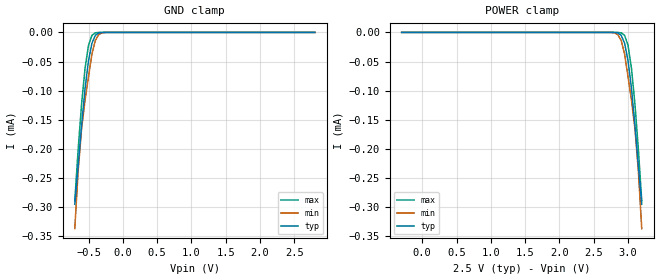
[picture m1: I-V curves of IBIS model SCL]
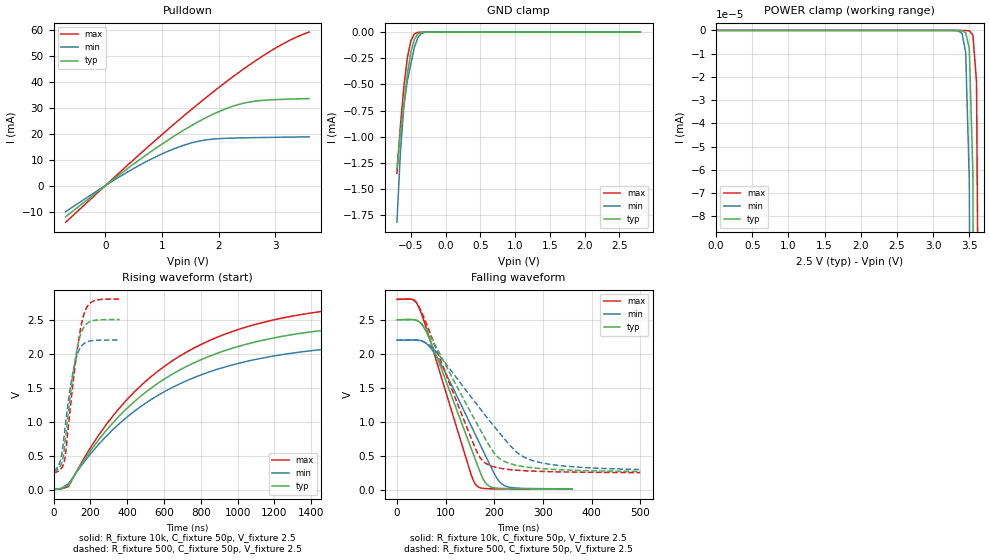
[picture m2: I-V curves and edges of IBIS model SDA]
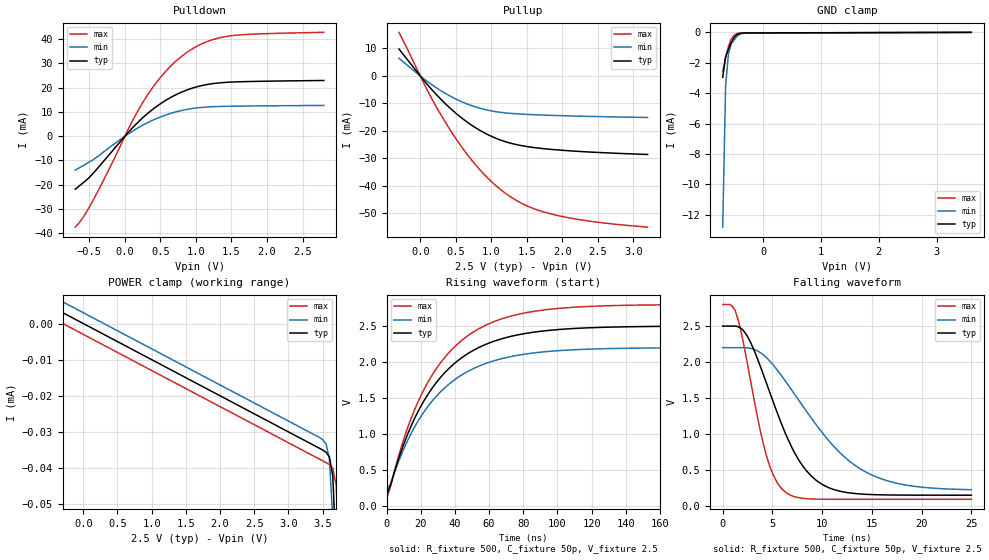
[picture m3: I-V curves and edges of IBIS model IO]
| PCA9538 - IBIS model
[IBIS Ver]   3.2
[Comment Char]   |_char
| VDD nom: 2.5v; min: 2.2v; max: 2.8v
[File name]   pca9538_2_5v.ibs
[File Rev]   1
[Date]   Aug 18, 2008 11:26:38 AM
[Source]
[Notes]
[Disclaimer]
(C) Copyright 2007 NXP Semiconductors
All rights reserved
NXP Semiconductors (NXP) does not warrant that this model and any other
accompanying information (Model) accurately or fully represents the
operating characteristics and specifications of the semiconductor
products to which the Model relates.  Moreover, the Model is furnished
on an "as is" and with "all faults" basis, and without support or
warranty of any kind.  NXP disclaims all warranties, whether expressed
or implied or statutory, including without limitation all implied
warranties of non-infringement, merchantability and fitness for any
purpose, and those arising from a course of dealing or usage of trade.
NXP does not convey any license under its or any third party's patents,
copyrights or other intellectual property or proprietary rights.
You and your company assume any and all risks and liability arising out
of the application or use of the Model.
In no event shall NXP be liable for any direct, indirect, special,
consequential or incidental damages, however caused, whether in
warranty, contract or tort (including negligence), strict liability or
other legal theory, including, without limitation, for lost profits,
business interruption, or corruption or loss of data or information,
arising out of or in connection with the use of or the inability to use
the Model, even if NXP has been advised of the possibility of such
damages.
NXP provides the Model as a courtesy to our customers. You and your
company shall not distribute, convey, sell, or give the Model to anyone
else without receiving prior written permission from NXP.
NXP reserves the right to make changes without notice to the Model to
improve reliability, function, or design.
Please be aware that your receipt and subsequent use of the Model shall
serve as acceptance of these terms and conditions.  If you do not
accept these terms, return or destroy the Model immediately.
[Copyright]
2008
| TSSOP16
[Component]   PCA9633PW
Si_location Pin
Timing_location Pin
[Manufacturer]   NXP Semiconductors
[Package]
R_pkg   3.92e-02   3.52e-02   4.56e-02
L_pkg   1.94n   1.65n   2.4n
C_pkg   0.446p   0.335p   0.771p
[Pin] signal_name   model_name   R_pin   L_pin   C_pin
1   A0   Addr   3.52E-02  2.40E-09  0.436E-12
2   A1   Addr   3.70E-02  1.93E-09  0.438E-12
3   RESETb   RESETb   4.56E-02  1.76E-09  0.345E-12
4   IO0   IO   4.00E-02  1.65E-09  0.335E-12
5   IO1   IO   4.00E-02  1.65E-09  0.335E-12
6   IO2   IO   4.56E-02  1.76E-09  0.345E-12
7   IO3   IO   3.70E-02  1.93E-09  0.438E-12
8   Vss   GND   3.52E-02  2.40E-09  0.452E-12
9   IO4   IO   3.52E-02  2.40E-09  0.452E-12
10   IO5   IO   3.70E-02  1.93E-09  0.438E-12
11   IO6   IO   4.56E-02  1.76E-09  0.345E-12
12   IO7   IO   4.00E-02  1.65E-09  0.771E-12
13   INTb   INT_OUT   4.00E-02  1.65E-09  0.771E-12
14   SCL   SCL   4.56E-02  1.76E-09  0.345E-12
15   SDA   SDA   3.70E-02  1.93E-09  0.438E-12
16   VDD   POWER   3.52E-02  2.40E-09  0.452E-12
| SO16
[Component]   PCA9633D16
Si_location Pin
Timing_location Pin
[Manufacturer]   NXP Semiconductors
[Package]
R_pkg   4.96e-02   3.94e-02   5.98e-02
L_pkg   2.52n   1.87n   3.16n
C_pkg   0.628p   0.494p   0.763p
[Pin] signal_name   model_name   R_pin   L_pin   C_pin
1   A0   Addr   5.98E-02  3.16E-09  7.63E-13
2   A1   Addr   4.55E-02  2.41E-09  6.04E-13
3   RESETb   RESETb   4.64E-02  1.93E-09  5.15E-13
4   IO0   IO   3.94E-02  1.87E-09  4.94E-13
5   IO1   IO   3.94E-02  1.87E-09  4.94E-13
6   IO2   IO   4.64E-02  1.93E-09  5.15E-13
7   IO3   IO   4.55E-02  2.41E-09  6.04E-13
8   Vss   GND   5.98E-02  3.16E-09  7.63E-13
9   IO4   IO   5.98E-02  3.16E-09  7.63E-13
10   IO5   IO   4.55E-02  2.41E-09  6.04E-13
11   IO6   IO   4.64E-02  1.93E-09  5.15E-13
12   IO7   IO   3.94E-02  1.87E-09  4.94E-13
13   INTb   INT_OUT   3.94E-02  1.87E-09  4.94E-13
14   SCL   SCL   4.64E-02  1.93E-09  5.15E-13
15   SDA   SDA   4.55E-02  2.41E-09  6.04E-13
16   VDD   POWER   5.98E-02  3.16E-09  7.63E-13
[Define Package Model]  HVQFN16
[Manufacturer]  ST-NXP Wireless
[OEM]  Unknown
[Description]  Full package model
|[Simulated] Chris Hunat
|[Approved] Wayne Nunn, Roger Real
[Number Of Pins]  16
[Pin Numbers]
|Pin Num   Terminal Name
1   | lead1:pin1
2   | lead2:pin2
3   | lead3:pin3
4   | lead4:pin4
5   | lead5:pin5
6   | lead6:pin6
7   | lead7:pin7
8   | lead8:pin8
9   | lead9:pin9
10   | lead10:pin10
11   | lead11:pin11
12   | lead12:pin12
13   | lead13:pin13
14   | lead14:pin14
15   | lead15:pin15
16   | lead16:pin16
[Model Data]
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[End Model Data]
[End Package Model]
| Models and submodels in the file (6): SCL (Input), SDA (I/O_open_drain), IO (I/O), RESETb (Input), INT_OUT (Open_drain), Addr (Input)
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[Model]   SCL
Model_type Input
Vinh=1.5
Vinl=0.75
C_comp   1.84p   1.81p   1.86p
[Temperature Range] 27   85   -40
[Voltage Range]   2.5   2.2   2.8
[GND Clamp]
-700mV    -295uA     -337uA     -289.5uA
-650mV    -228.6uA   -236.2uA   -199.5uA
-600mV    -158.8uA   -164.3uA   -122uA
-550mV    -96.13uA   -116.2uA   -61.46uA
-500mV    -48.62uA   -75.94uA   -22.35uA
-450mV    -18.67uA   -37.44uA   -5.001uA
-400mV    -4.926uA   -13.83uA   -710.6nA
-350mV    -920.5nA   -3.647uA   -77.67nA
-300mV    -138.4nA   -722.3nA   -7.551nA
-200mV    -2.42nA    -18.61nA   -62.47pA
2.8V      6.71pA     20.63pA    5.609pA
[POWER Clamp]
-300mV    6.71pA     20.63pA    5.609pA
2.7V      -2.42nA    -18.61nA   -62.47pA
2.8V      -138.4nA   -722.3nA   -7.551nA
2.85V     -920.5nA   -3.647uA   -77.68nA
2.9V      -4.926uA   -13.83uA   -710.6nA
2.95V     -18.67uA   -37.44uA   -5.001uA
3V        -48.62uA   -75.94uA   -22.35uA
3.05V     -96.13uA   -116.2uA   -61.46uA
3.1V      -158.8uA   -164.3uA   -122uA
3.15V     -228.6uA   -236.2uA   -199.5uA
3.2V      -295uA     -337uA     -289.5uA
[Model]   SDA
Model_type I/O_open_drain
Enable Active-High
Vinh=1.75
Vinl=0.75
Vref=2.5
Vmeas=1.25
Rref=10k
Cref=50p
C_comp   6.2p   6p   6.4p
[Temperature Range] 27   85   -40
[Voltage Range]   2.5   2.2   2.8
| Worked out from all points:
|   slope of the pulldown table from 0 to 0.375 V, typ, clamps not added: 59.7 ohm
|   GND clamp passes 1 mA (typ) near -0.65 V on its own axis
|   falling waveform, R_fixture 10k, C_fixture 50p, V_fixture 2.5: 20-80 % time 78.3ns typ, 88.6ns min, 71.3ns max; typ from 2.5 V to 0.016 V
|   falling waveform, R_fixture 500, C_fixture 50p, V_fixture 2.5: 20-80 % time 100ns typ, 125ns min, 83.5ns max; typ from 2.5 V to 0.275 V
|   rising waveform, R_fixture 10k, C_fixture 50p, V_fixture 2.5: 20-80 % time 701ns typ, 702ns min, 701ns max; typ from 0.015 V to 2.5 V
|   rising waveform, R_fixture 500, C_fixture 50p, V_fixture 2.5: 20-80 % time 63.7ns typ, 60.2ns min, 67.6ns max; typ from 0.265 V to 2.5 V
[Pulldown]
-700mV    -12mA      -10.04mA   -14.1mA
200mV     3.382mA    2.732mA    4.024mA
800mV     13.01mA    10.12mA    15.83mA
1.35V     20.92mA    15.31mA    26.22mA
1.6V      24.11mA    16.9mA     30.76mA
1.85V     26.97mA    17.83mA    35.17mA
2.2V      30.21mA    18.29mA    41.08mA
2.55V     32.25mA    18.47mA    46.6mA
2.85V     32.97mA    18.58mA    50.94mA
3.15V     33.27mA    18.68mA    54.79mA
3.4V      33.44mA    18.75mA    57.48mA
3.6V      33.55mA    18.8mA     59.2mA
[GND Clamp]
-700mV    -1.302mA   -1.818mA   -1.351mA
-650mV    -970uA     -1.147mA   -895.5uA
-600mV    -683.7uA   -711.2uA   -519.4uA
-550mV    -399.4uA   -467.3uA   -244.7uA
-500mV    -192.3uA   -305.3uA   -82.59uA
-450mV    -70.46uA   -146.9uA   -17.18uA
-400mV    -17.84uA   -52.38uA   -2.302uA
-350mV    -3.222uA   -13.43uA   -238.8nA
-300mV    -468.9nA   -2.601uA   -22.09nA
-200mV    -7.684nA   -64.03nA   -166.2pA
2.8V      13.86pA    54.83pA    11.22pA
[POWER Clamp]
0V        16.1pA     60.18pA    13.22pA
3.35V     -12.07pA   -161.9pA   -287.6fA
3.4V      -112.6pA   -1.322nA   -1.543pA
3.45V     -940.4pA   -9.345nA   -14.46pA
3.5V      -7.684nA   -64.03nA   -166.2pA
3.55V     -61.43nA   -424.5nA   -1.939nA
3.6V      -468.9nA   -2.601uA   -22.09nA
3.65V     -3.222uA   -13.43uA   -238.8nA
4V        -1.302mA   -1.818mA   -1.351mA
[Falling Waveform]
R_fixture=10k
C_fixture=50p
V_fixture=2.5
V_fixture_min=2.2
V_fixture_max=2.8
0s        2.5V       2.2V       2.8V
32.73ns   2.503V     2.203V     2.797V
47.27ns   2.46V      2.196V     2.646V
83.64ns   1.925V     1.936V     1.836V
152.7ns   607.1mV    940.1mV    222.7mV
163.6ns   400.2mV    777.2mV    65.93mV
185.5ns   80mV       453mV      21.86mV
207.3ns   27.97mV    155.1mV    18.26mV
221.8ns   23.24mV    63.63mV    17.19mV
360ns     16.11mV    18.89mV    14.52mV
[Falling Waveform]
R_fixture=500
C_fixture=50p
V_fixture=2.5
V_fixture_min=2.2
V_fixture_max=2.8
0s        2.5V       2.2V       2.8V
30.3ns    2.502V     2.202V     2.8V
45.45ns   2.473V     2.197V     2.691V
80.81ns   2.098V     2.027V     2.071V
161.6ns   1.01V      1.28V      606mV
181.8ns   749.8mV    1.095V     397mV
212.1ns   457.4mV    826.1mV    321.3mV
247.5ns   361.6mV    549.7mV    292mV
272.7ns   332.9mV    448.7mV    281.5mV
500ns     274.6mV    303.4mV    257.5mV
[Rising Waveform]
R_fixture=10k
C_fixture=50p
V_fixture=2.5
V_fixture_min=2.2
V_fixture_max=2.8
0s        14.58mV    15.74mV    13.8mV
80.81ns   70.46mV    91.25mV    51.11mV
202ns     580.6mV    534.6mV    627.3mV
323.2ns   988.5mV    888.1mV    1.089V
565.7ns   1.563V     1.386V     1.74V
808.1ns   1.919V     1.695V     2.143V
1.131us   2.193V     1.933V     2.453V
1.495us   2.35V      2.07V      2.631V
2.02us    2.447V     2.154V     2.74V
4us       2.498V     2.199V     2.798V
[Rising Waveform]
R_fixture=500
C_fixture=50p
V_fixture=2.5
V_fixture_min=2.2
V_fixture_max=2.8
0s        265.3mV    283.1mV    253.4mV
40ns      369.1mV    459mV      309.9mV
50.91ns   463.1mV    641.2mV    356.2mV
61.82ns   677.4mV    888.7mV    463.3mV
90.91ns   1.385V     1.494V     1.201V
120ns     1.948V     1.904V     1.881V
145.5ns   2.265V     2.085V     2.345V
170.9ns   2.412V     2.157V     2.622V
221.8ns   2.487V     2.194V     2.775V
360ns     2.5V       2.2V       2.8V
[Ramp]
R_load=500
dV/dt_r   1.769E+0/6.440E-8   1.721E+0/6.204E-8   1.801E+0/6.654E-8
dV/dt_f   1.737E+0/1.304E-7   1.574E+0/1.747E-7   1.791E+0/9.775E-8
|[End   SDA
[Model]   IO
Model_type I/O
Enable Active-High
Polarity Non-Inverting
Vinh=1.5
Vinl=0.75
Vref=2.5
Vmeas=1.25
Rref=500
Cref=50p
C_comp   8p   7.8p   8.2p
[Temperature Range] 27   85   -40
[Voltage Range]   2.5   2.2   2.8
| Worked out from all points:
|   slope of the pulldown table from 0 to 0.375 V, typ, clamps not added: 35.1 ohm
|   slope of the pullup table from 0 to 0.375 V, typ, clamps not added: 35.3 ohm
|   GND clamp passes 1 mA (typ) near -0.59 V on its own axis
|   falling waveform, R_fixture 500, C_fixture 50p, V_fixture 2.5: 20-80 % time 4.19ns typ, 6.82ns min, 2.45ns max; typ from 2.5 V to 0.148 V
|   rising waveform, R_fixture 500, C_fixture 50p, V_fixture 2.5: 20-80 % time 35.7ns typ, 35.9ns min, 35.6ns max; typ from 0.148 V to 2.5 V
[Pullup]
-300mV    9.769mA    6.423mA    15.84mA
150mV     -4.623mA   -2.955mA   -7.715mA
450mV     -12.42mA   -7.741mA   -20.8mA
600mV     -15.62mA   -9.577mA   -26.43mA
800mV     -19.18mA   -11.46mA   -32.96mA
950mV     -21.32mA   -12.45mA   -37.11mA
1.15V     -23.49mA   -13.3mA    -41.69mA
1.45V     -25.46mA   -13.91mA   -46.59mA
1.65V     -26.19mA   -14.16mA   -48.73mA
1.85V     -26.72mA   -14.35mA   -50.23mA
2.4V      -27.68mA   -14.73mA   -52.84mA
3.2V      -28.55mA   -15.1mA    -54.96mA
[Pulldown]
-700mV    -21.86mA   -13.96mA   -37.51mA
-600mV    -19.49mA   -12.35mA   -33.95mA
-450mV    -15.4mA    -9.754mA   -26.53mA
-200mV    -6.877mA   -4.259mA   -12.24mA
100mV     3.26mA     1.947mA    5.975mA
250mV     7.594mA    4.531mA    13.84mA
500mV     13.39mA    7.941mA    24.26mA
800mV     18.21mA    10.62mA    32.99mA
1.1V      20.99mA    11.92mA    38.33mA
1.4V      22.16mA    12.31mA    40.99mA
1.8V      22.58mA    12.47mA    42.08mA
2.8V      22.98mA    12.69mA    42.84mA
[GND Clamp]
-700mV    -2.949mA   -12.82mA   -2.591mA
-650mV    -1.618mA   -3.556mA   -1.65mA
-600mV    -1.097mA   -1.385mA   -902.1uA
-550mV    -647.3uA   -748.9uA   -419uA
-500mV    -317.7uA   -474.1uA   -166.2uA
-450mV    -139.5uA   -244.4uA   -69.6uA
-400mV    -64.91uA   -109.4uA   -44.89uA
-350mV    -42.27uA   -54.37uA   -40.06uA
-250mV    -35.59uA   -33.25uA   -38.46uA
3.6V      2.994uA    5.987uA    -359.9pA
[POWER Clamp]
-300mV    2.994uA    5.987uA    -359.9pA
3.5V      -34.97uA   -32.08uA   -37.95uA
3.55V     -35.59uA   -33.25uA   -38.46uA
3.6V      -36.9uA    -37.47uA   -39.01uA
3.65V     -42.27uA   -54.37uA   -40.06uA
3.7V      -64.91uA   -109.4uA   -44.89uA
3.75V     -139.5uA   -244.4uA   -69.59uA
4V        -2.949mA   -12.82mA   -2.591mA
[Falling Waveform]
R_fixture=500
C_fixture=50p
V_fixture=2.5
V_fixture_min=2.2
V_fixture_max=2.8
0s        2.5V       2.2V       2.8V
1.263ns   2.499V     2.2V       2.714V
2.525ns   2.349V     2.196V     1.946V
4.545ns   1.65V      2.041V     629.2mV
6.313ns   1.004V     1.733V     190.3mV
7.828ns   598.5mV    1.432V     109.2mV
9.343ns   361.2mV    1.139V     94.03mV
14.14ns   162.4mV    489.8mV    90.74mV
18.18ns   149.6mV    295.1mV    90.73mV
25ns      148.3mV    224.8mV    90.73mV
[Rising Waveform]
R_fixture=500
C_fixture=50p
V_fixture=2.5
V_fixture_min=2.2
V_fixture_max=2.8
0s        148.2mV    216.3mV    90.72mV
2.424ns   292.1mV    307.3mV    278.2mV
7.273ns   669.8mV    629.9mV    711.5mV
12.12ns   983.1mV    897.6mV    1.071V
24.24ns   1.551V     1.384V     1.72V
38.79ns   1.96V      1.735V     2.188V
58.18ns   2.247V     1.981V     2.513V
80ns      2.392V     2.106V     2.678V
109.1ns   2.465V     2.17V      2.761V
240ns     2.5V       2.2V       2.8V
[Ramp]
R_load=500
dV/dt_r   6.958E-3/1.622E-9   5.948E-3/1.898E-9   8.071E-3/1.411E-9
dV/dt_f   1.411E+0/5.668E-10   1.190E+0/1.129E-9   1.626E+0/2.812E-10
|[End   IO
